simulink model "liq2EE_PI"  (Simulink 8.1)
settings: Solver=ode45  StartTime=0.0  StopTime=500  FixedStep=1  RelTol=1e-6
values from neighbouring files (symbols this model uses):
  a = log(spiralfactor)*2/pi    [nyqlog.m]    (also in para2nl.m = k12/(2*Ar*sqrt(h1b-h2b)); para2nl_PI.m = k12/(2*Ar*sqrt(h1b-h2b)); PrPara2nl_PI.m = k12/(2*Ar*sqrt(h1b-h2b)))
  Ar = 6*25.4    (= 152.4)    [para2nl.m]    (also in para2nl_PI.m; PrPara2nl_PI.m)
  b = k2/(2*Ar*sqrt(h2b))    [para2nl.m]    (also in para2nl_PI.m; PrPara2nl_PI.m)
  K = acker(A,B,[p p])    [para2nl.m]    (also in para2nl_PI.m = acker(Aa,Ba,[p,p,p]); PrPara2nl_PI.m = acker(Aa,Ba,[p,p,p]); TestesEE.m = acker(A,B,[p,-.6-1.02i,-.6+1.02i]); TestesEEobsPert.m = acker(A,B,[p,-.6-1.0198i,-.6+1.0198i]))
  k1 = 0    [para2nl.m]    (also in para2nl_PI.m; PrPara2nl_PI.m)
  k12 = 38    [para2nl.m]    (also in para2nl_PI.m; PrPara2nl_PI.m)
  k2 = 11.5    [para2nl.m]    (also in para2nl_PI.m; PrPara2nl_PI.m)
  Ki = -K(3)    [para2nl_PI.m]    (also in PrPara2nl_PI.m; TestesEEcanalI.m = Ka(1),K=Ka(2:4),)
  Kp = -Ki/p    [para2nl_PI.m]    (also in PrPara2nl_PI.m)
  L = L'    [para2nl.m]    (also in para2nl_PI.m; PrPara2nl_PI.m; TestesEE.m; TestesEEcanalI.m)
  qmax = 90    [para2nl.m]    (also in para2nl_PI.m; PrPara2nl_PI.m)
  qmin = -85    [para2nl.m]    (also in para2nl_PI.m; PrPara2nl_PI.m)
libraries: simulink x2

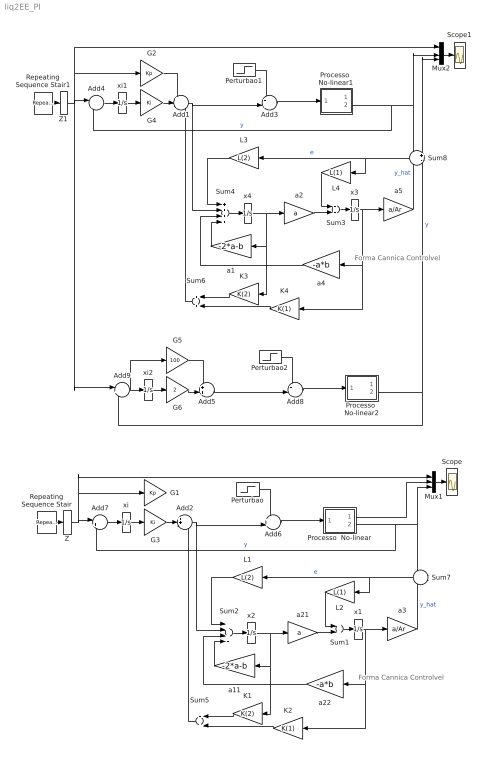
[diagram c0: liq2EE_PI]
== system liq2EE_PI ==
  note: Forma Cannica Controlvel
  note: Forma Cannica Controlvel
  Add1 : Sum  Inputs=++-
  Add2 : Sum  Inputs=++-
  Add{3,5..6,8} (4 alike) : Sum  Inputs=++|
  Add4 : Sum  Inputs=|+-
  Add7 : Sum  Inputs=|+-
  Add9 : Sum  Inputs=|+-
  G1 : Gain  Gain=Kp
  G2 : Gain  Gain=Kp
  G3 : Gain  Gain=Ki
  G4 : Gain  Gain=Ki
  G5 : Gain  Gain=100
  G6 : Gain  Gain=2
  K1 : Gain  Gain=K(2)
  K2 : Gain  Gain=K(1)
  K3 : Gain  Gain=K(2)
  K4 : Gain  Gain=K(1)
  L1 : Gain  Gain=L(2)
  L2 : Gain  Gain=L(1)
  L3 : Gain  Gain=L(2)
  L4 : Gain  Gain=L(1)
  Mux1 : Mux  Inputs=3
  Mux2 : Mux
  Perturbao : Step  Time=350  After=50  SampleTime=0
  Perturbao1 : Step  Time=350  After=50  SampleTime=0
  Perturbao2 : Step  Time=350  After=50  SampleTime=0
  Processo  No-linear : Subsystem
  Processo  No-linear1 : Subsystem
  Processo  No-linear2 : Subsystem
  Repeating Sequence Stair : simulink/Sources/Repeating Sequence Stair  OutValues=[2 5 12 5 2].'  tsamp=100  OutMin=[]  OutMax=[]  OutDataTypeStr=double  OutputDataTypeScalingMode=double  OutDataType=fixdt(0,8)  ConRadixGroup=Best Precision: Vector-wise  OutScaling=2^-12
  Repeating Sequence Stair1 : simulink/Sources/Repeating Sequence Stair  OutValues=[2 5 12 5 2].'  tsamp=100  OutMin=[]  OutMax=[]  OutDataTypeStr=double  OutputDataTypeScalingMode=double  OutDataType=fixdt(0,8)  ConRadixGroup=Best Precision: Vector-wise  OutScaling=2^-12
  Scope : Scope
  Scope1 : Scope
  Sum{1,3,5..6} (4 alike) : Sum
  Sum2 : Sum  Inputs=++++
  Sum4 : Sum  Inputs=++++
  Sum7 : Sum  Inputs=+-
  Sum8 : Sum  Inputs=+-
  Z : ZeroOrderHold
  Z1 : ZeroOrderHold
  a1 : Gain  Gain=-2*a-b
  a11 : Gain  Gain=-2*a-b
  a2 : Gain  Gain=a
  a21 : Gain  Gain=a
  a22 : Gain  Gain=-a*b
  a3 : Gain  Gain=a/Ar
  a4 : Gain  Gain=-a*b
  a5 : Gain  Gain=a/Ar
  x{1..4} (4 alike) : Integrator
  xi : Integrator
  xi1 : Integrator
  xi2 : Integrator
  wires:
  Mux1/1 -> Scope/1
  x2/1 -> a21/1, a11/1, K1/1
  Sum2/1 -> x2/1
  x1/1 -> a22/1, K2/1, a3/1
  Sum1/1 -> x1/1
  Add2/1 -> Sum2/2, Add6/2
  Processo  No-linear/2(H2) -> Mux1/3, Sum7/1, Add7/2  "y"
  L1/1 -> Sum2/1
  K1/1 -> Sum5/1
  K2/1 -> Sum5/2
  Sum7/1 -> L1/1, L2/1  "e"
  a11/1 -> Sum2/4
  a22/1 -> Sum2/3
  a3/1 -> Sum7/2  "y_hat"
  Processo  No-linear/1(H1) -> Mux1/2
  a21/1 -> Sum1/2
  L2/1 -> Sum1/1
  Perturbao/1 -> Add6/1
  Add6/1 -> Processo  No-linear/1(u)
  xi/1 -> G3/1
  Add7/1 -> xi/1
  Sum5/1 -> Add2/3
  G3/1 -> Add2/2
  Repeating Sequence Stair/1 -> Z/1
  Z/1 -> Add7/1, G1/1, Mux1/1
  Mux2/1 -> Scope1/1
  x4/1 -> a2/1, a1/1, K3/1
  Sum4/1 -> x4/1
  x3/1 -> a4/1, K4/1, a5/1
  Sum3/1 -> x3/1
  Add1/1 -> Sum4/2, Add3/2
  Processo  No-linear1/2(H2) -> Mux2/3, Sum8/1, Add4/2  "y"
  L3/1 -> Sum4/1
  K3/1 -> Sum6/1
  K4/1 -> Sum6/2
  Sum8/1 -> L3/1, L4/1  "e"
  a1/1 -> Sum4/4
  a4/1 -> Sum4/3
  a5/1 -> Sum8/2  "y_hat"
  a2/1 -> Sum3/2
  L4/1 -> Sum3/1
  Perturbao1/1 -> Add3/1
  Add3/1 -> Processo  No-linear1/1(u)
  xi1/1 -> G4/1
  Add4/1 -> xi1/1
  Sum6/1 -> Add1/3
  G4/1 -> Add1/2
  Repeating Sequence Stair1/1 -> Z1/1
  G2/1 -> Add1/1
  Add5/1 -> Add8/2
  Processo  No-linear2/2(H2) -> Add9/2, Mux2/4  "y"
  Perturbao2/1 -> Add8/1
  Add8/1 -> Processo  No-linear2/1(u)
  xi2/1 -> G6/1
  Add9/1 -> G5/1, xi2/1
  G6/1 -> Add5/2
  Z1/1 -> G2/1, Mux2/1, Add9/1, Add4/1
  G5/1 -> Add5/1

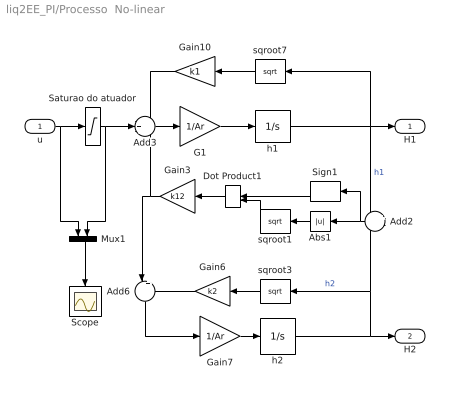
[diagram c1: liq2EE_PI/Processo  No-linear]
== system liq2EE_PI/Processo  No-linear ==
  u : Inport
  Abs1 : Abs
  Add2 : Sum  Inputs=+-
  Add3 : Sum  Inputs=-+-
  Add6 : Sum  Inputs=|+-
  Dot Product1 : DotProduct
  G1 : Gain  Gain=1/Ar
  Gain10 : Gain  Gain=k1
  Gain3 : Gain  Gain=k12
  Gain6 : Gain  Gain=k2
  Gain7 : Gain  Gain=1/Ar
  Mux1 : Mux  Inputs=2
  Saturao do atuador : Saturate  UpperLimit=qmax  LowerLimit=qmin
  Scope : Scope
  Sign1 : Signum
  h1 : Integrator  LimitOutput=on  UpperSaturationLimit=16.5  LowerSaturationLimit=0
  h2 : Integrator  LimitOutput=on  UpperSaturationLimit=16.5  LowerSaturationLimit=0
  sqroot1 : Math  Operator=sqrt
  sqroot3 : Math  Operator=sqrt
  sqroot7 : Math  Operator=sqrt
  H1 : Outport
  H2 : Outport  Port=2
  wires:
  h1/1 -> Add2/1, H1/1, sqroot7/1  "h1"
  h2/1 -> Add2/2, sqroot3/1, H2/1  "h2"
  Saturao do atuador/1 -> Add3/2, Mux1/2
  Add6/1 -> Gain7/1
  Gain10/1 -> Add3/1
  sqroot7/1 -> Gain10/1
  Gain6/1 -> Add6/2
  Gain7/1 -> h2/1
  sqroot3/1 -> Gain6/1
  G1/1 -> h1/1
  Gain3/1 -> Add6/1, Add3/3
  Add3/1 -> G1/1
  Dot Product1/1 -> Gain3/1
  sqroot1/1 -> Dot Product1/2
  Sign1/1 -> Dot Product1/1
  Abs1/1 -> sqroot1/1
  Add2/1 -> Abs1/1, Sign1/1
  u/1 -> Saturao do atuador/1, Mux1/1
  Mux1/1 -> Scope/1

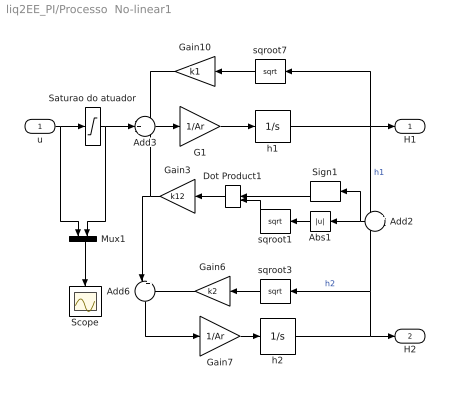
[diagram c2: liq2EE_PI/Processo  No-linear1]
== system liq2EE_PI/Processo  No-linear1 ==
  u : Inport
  Abs1 : Abs
  Add2 : Sum  Inputs=+-
  Add3 : Sum  Inputs=-+-
  Add6 : Sum  Inputs=|+-
  Dot Product1 : DotProduct
  G1 : Gain  Gain=1/Ar
  Gain10 : Gain  Gain=k1
  Gain3 : Gain  Gain=k12
  Gain6 : Gain  Gain=k2
  Gain7 : Gain  Gain=1/Ar
  Mux1 : Mux  Inputs=2
  Saturao do atuador : Saturate  UpperLimit=qmax  LowerLimit=qmin
  Scope : Scope
  Sign1 : Signum
  h1 : Integrator  LimitOutput=on  UpperSaturationLimit=16.5  LowerSaturationLimit=0
  h2 : Integrator  LimitOutput=on  UpperSaturationLimit=16.5  LowerSaturationLimit=0
  sqroot1 : Math  Operator=sqrt
  sqroot3 : Math  Operator=sqrt
  sqroot7 : Math  Operator=sqrt
  H1 : Outport
  H2 : Outport  Port=2
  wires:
  h1/1 -> Add2/1, H1/1, sqroot7/1  "h1"
  h2/1 -> Add2/2, sqroot3/1, H2/1  "h2"
  Saturao do atuador/1 -> Add3/2, Mux1/2
  Add6/1 -> Gain7/1
  Gain10/1 -> Add3/1
  sqroot7/1 -> Gain10/1
  Gain6/1 -> Add6/2
  Gain7/1 -> h2/1
  sqroot3/1 -> Gain6/1
  G1/1 -> h1/1
  Gain3/1 -> Add6/1, Add3/3
  Add3/1 -> G1/1
  Dot Product1/1 -> Gain3/1
  sqroot1/1 -> Dot Product1/2
  Sign1/1 -> Dot Product1/1
  Abs1/1 -> sqroot1/1
  Add2/1 -> Abs1/1, Sign1/1
  u/1 -> Saturao do atuador/1, Mux1/1
  Mux1/1 -> Scope/1

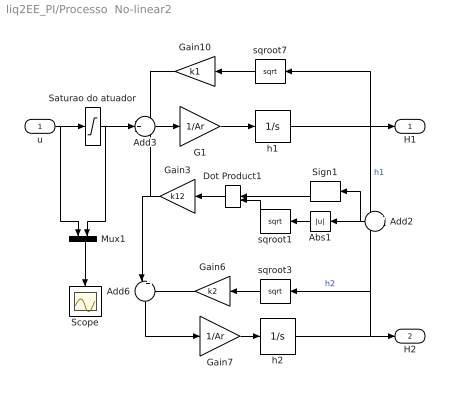
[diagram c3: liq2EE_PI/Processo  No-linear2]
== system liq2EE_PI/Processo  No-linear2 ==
  u : Inport
  Abs1 : Abs
  Add2 : Sum  Inputs=+-
  Add3 : Sum  Inputs=-+-
  Add6 : Sum  Inputs=|+-
  Dot Product1 : DotProduct
  G1 : Gain  Gain=1/Ar
  Gain10 : Gain  Gain=k1
  Gain3 : Gain  Gain=k12
  Gain6 : Gain  Gain=k2
  Gain7 : Gain  Gain=1/Ar
  Mux1 : Mux  Inputs=2
  Saturao do atuador : Saturate  UpperLimit=qmax  LowerLimit=qmin
  Scope : Scope
  Sign1 : Signum
  h1 : Integrator  LimitOutput=on  UpperSaturationLimit=16.5  LowerSaturationLimit=0
  h2 : Integrator  LimitOutput=on  UpperSaturationLimit=16.5  LowerSaturationLimit=0
  sqroot1 : Math  Operator=sqrt
  sqroot3 : Math  Operator=sqrt
  sqroot7 : Math  Operator=sqrt
  H1 : Outport
  H2 : Outport  Port=2
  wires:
  h1/1 -> Add2/1, H1/1, sqroot7/1  "h1"
  h2/1 -> Add2/2, sqroot3/1, H2/1  "h2"
  Saturao do atuador/1 -> Add3/2, Mux1/2
  Add6/1 -> Gain7/1
  Gain10/1 -> Add3/1
  sqroot7/1 -> Gain10/1
  Gain6/1 -> Add6/2
  Gain7/1 -> h2/1
  sqroot3/1 -> Gain6/1
  G1/1 -> h1/1
  Gain3/1 -> Add6/1, Add3/3
  Add3/1 -> G1/1
  Dot Product1/1 -> Gain3/1
  sqroot1/1 -> Dot Product1/2
  Sign1/1 -> Dot Product1/1
  Abs1/1 -> sqroot1/1
  Add2/1 -> Abs1/1, Sign1/1
  u/1 -> Saturao do atuador/1, Mux1/1
  Mux1/1 -> Scope/1
